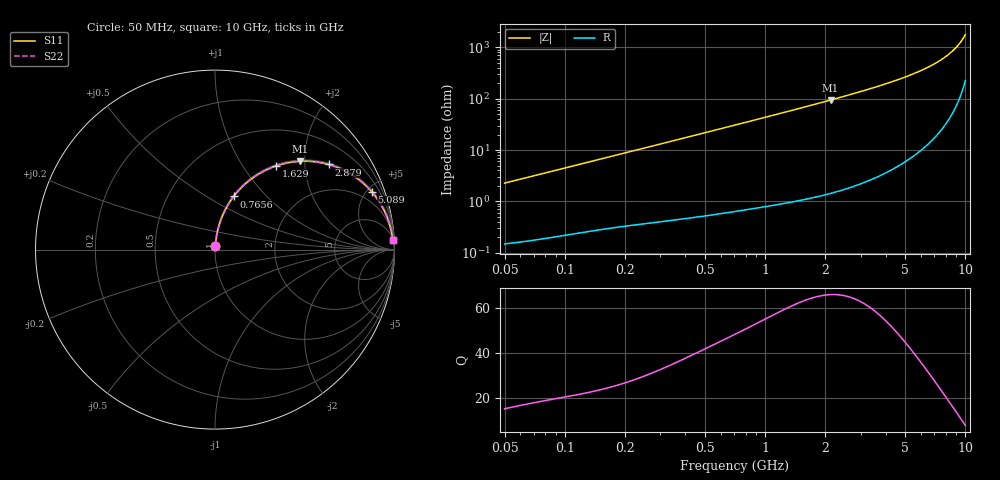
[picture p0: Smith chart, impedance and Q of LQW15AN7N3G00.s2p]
!Murata Part Number: LQW15AN7N3G00
!These Parameters are Measured in Series Mode Connection
!  o--[Z]--o
!Port1  Port2
!  o-------o
!Freq. Start=50[MHz] Stop=10[GHz], 401[Steps]
# Hz S RI R 50
!Freq.(Hz)	S 11(Real)	S 11(Imag)	S 21(Real)	S 21(Imag)	S 12(Real)	S 12(Imag)	S 22(Real)	S 22(Imag)
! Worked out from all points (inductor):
!   401 points, 50 MHz to 10 GHz, reference 50 ohm
!   read as one part in series: L = 7.18 nH near 51.34 MHz
!   highest Q = 66.1 at 2.123 GHz (marker M1), where L = 7.08 nH
!   S11 on the Smith chart (normalised r, x): 50 MHz: 1.00, +0.05; 765.6 MHz: 1.01, +0.67; 1.629 GHz: 1.02, +1.43; 2.879 GHz: 1.04, +2.64; 5.089 GHz: 1.12, +5.44; 10 GHz: 6, +36
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5e7  0.00199 0.0226  0.998 -0.0226  0.998 -0.0226  0.00199 0.0226
1.214486e8  0.00535 0.0537  0.9946 -0.0537  0.9946 -0.0537  0.00535 0.0537
2.949953e8  0.0202 0.126  0.9798 -0.126  0.9798 -0.126  0.0202 0.126
4.81571e8  0.0465 0.1989  0.9535 -0.1989  0.9535 -0.1989  0.0465 0.1989
7.071068e8  0.091 0.2775  0.909 -0.2775  0.909 -0.2775  0.091 0.2775
7.655974e8  0.1044 0.2959  0.8956 -0.2959  0.8956 -0.2959  0.1044 0.2959
1.124152e9  0.1974 0.3894  0.8026 -0.3894  0.8026 -0.3894  0.1974 0.3894
1.628911e9  0.3408 0.4662  0.6592 -0.4662  0.6592 -0.4662  0.3408 0.4662
1.717543e9  0.3655 0.4739  0.6345 -0.4739  0.6345 -0.4739  0.3655 0.4739
2.122994e9  0.472 0.4917  0.528 -0.4917  0.528 -0.4917  0.472 0.4917
2.879108e9  0.6332 0.4742  0.3668 -0.4742  0.3668 -0.4742  0.6332 0.4742
3.420121e9  0.7187 0.4413  0.2813 -0.4413  0.2813 -0.4413  0.7187 0.4413
4.171863e9  0.8053 0.3866  0.1947 -0.3866  0.1947 -0.3866  0.8053 0.3866
5.088839e9  0.8754 0.3191  0.1246 -0.3191  0.1246 -0.3191  0.8754 0.3191
6.458996e9  0.9365 0.2287  0.0635 -0.2287  0.0635 -0.2287  0.9365 0.2287
7.086521e9  0.9539 0.1922  0.0461 -0.1922  0.0461 -0.1922  0.9539 0.1922
7.775012e9  0.9678 0.1553  0.0322 -0.1553  0.0322 -0.1553  0.9678 0.1553
8.307378e9  0.9758 0.1288  0.0242 -0.1288  0.0242 -0.1288  0.9758 0.1288
8.876195e9  0.9822 0.1022  0.0178 -0.1022  0.0178 -0.1022  0.9822 0.1022
9.236013e9  0.9854 0.0863  0.0146 -0.0863  0.0146 -0.0863  0.9854 0.0863
9.738562e9  0.9887 0.065  0.0113 -0.065  0.0113 -0.065  0.9887 0.065
1e10  0.99 0.0544  0.00998 -0.0544  0.00998 -0.0544  0.99 0.0544
